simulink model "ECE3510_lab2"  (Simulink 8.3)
settings: Solver=ode1  StartTime=0.0  StopTime=Inf  FixedStep=Ts  RelTol=1e-3
PostLoadFcn:
  | , if any(exist('dsrtsu_mdlpostloadfcn', 'file') == [2, 3, 6]), try dsrtsu_mdlpostloadfcn('Execute', bdroot); catch fprintf('Error in PostLoadFcn (dsrtsu_mdlpostloadfcn) for model "%s":
  |  %s
  | ', bdroot, lasterr); end, end,
InitFcn:
  | Ts=1e-4;
  | nd=30;
libraries: rtilib1104 x4

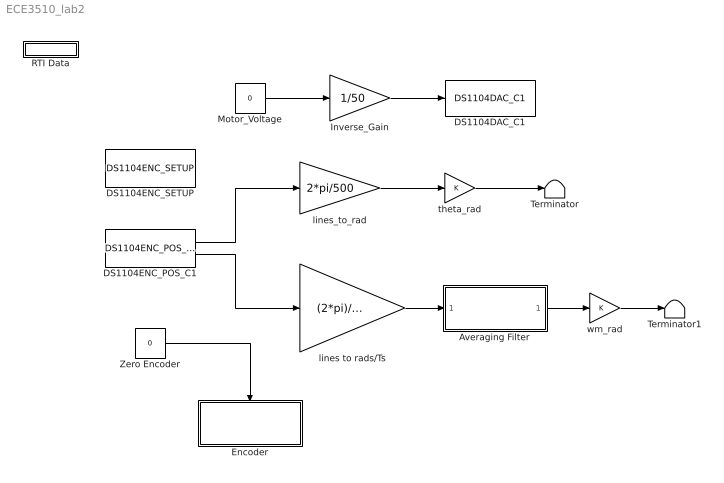
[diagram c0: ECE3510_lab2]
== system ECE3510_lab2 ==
  Averaging Filter : Subsystem
  DS1104DAC_C1 : rtilib1104/DS1104 MASTER PPC/DS1104DAC_C1  ChannelNo=1  InitValue=0  TermMode=0  TermValue=0  Reserved1=[]  Reserved2=[]  Reserved3=[]  Reserved4=[]  DialogFcn=gui1104dac  UnitName={ 'DS1104DAC_C'}  UnitValues={ 1 }  DSProperties=struct('RTI',struct('Version',uint32(1),'BlockType',struct('isSLSource',uint8(0),'isSLSink',uint8(1),'isHWSource',uint8(0),'isHWSink',uint8(1),'isSetup',uint8(0),'isInline',uint8(1),'isNonInline',uint8(0),'isInterrupt',uint8(0),'isChannelwise',uint8(1)),'IOBoardType','DS1104MASTER','UnitType','DAC','Identifier','DAC','DialogType','ML','BlockSet','NONE','SlaveProcessor','NONE'))
  DS1104ENC_POS_C1 : rtilib1104/DS1104 MASTER PPC/DS1104ENC_POS_C1  ChannelNo=1  PosValue=0  Reserved1=[]  Reserved2=[]  Reserved3=[]  Reserved4=[]  DialogFcn=gui1104enc_pos  UnitName={'DS1104ENC_POS_C'}  UnitValues={ 1 }  DSProperties=struct('RTI',struct('Version',uint32(1),'BlockType',struct('isSLSource',uint8(1),'isSLSink',uint8(0),'isHWSource',uint8(1),'isHWSink',uint8(0),'isSetup',uint8(0),'isInline',uint8(1),'isNonInline',uint8(0),'isInterrupt',uint8(0),'isChannelwise',uint8(1)),'IOBoardType','DS1104MASTER','UnitType','ENC','Identifier','ENCPOSCH','DialogType','ML','BlockSet','NONE','SlaveProcessor','NONE'))
  DS1104ENC_SETUP : rtilib1104/DS1104 MASTER PPC/DS1104ENC_SETUP  Reserved1=[]  Reserved2=[]  Reserved3=[]  Reserved4=[]  DialogFcn=gui1104enc_setup  UnitName={'DS1104ENC_SETUP'}  UnitValues={ [] }  DSProperties=struct('RTI',struct('Version',uint32(1),'BlockType',struct('isSLSource',uint8(0),'isSLSink',uint8(0),'isHWSource',uint8(0),'isHWSink',uint8(0),'isSetup',uint8(0),'isInline',uint8(1),'isNonInline',uint8(0),'isInterrupt',uint8(0),'isChannelwise',uint8(0)),'IOBoardType','DS1104MASTER','UnitType','ENC','Identifier','ENCSETUP','DialogType','ML','BlockSet','NONE','SlaveProcessor','NONE'))
  Encoder : Subsystem
  Inverse_Gain : Gain  Gain=1/50
  Motor_Voltage : Constant  Value=0
  RTI Data : Subsystem  Tag=struct('RTIDataServer',struct('RTIDataServerVs','2','RTIModelDescription','struct(''main'',''ECE3510_lab2'',''sub'','''',''isMp'',0)'))  LoadFcn="if exist('rtidc'), try,  rtidc('DataHostBlockClbLoad', gcbh); catch, disp(['Warning: ''LoadFcn'' for RTI Data block failed: ' lasterr]); end, end,"
  Terminator : Terminator
  Terminator1 : Terminator
  Zero Encoder : Constant  Value=0
  lines to rads/Ts : Gain  Gain=(2*pi)/(500*Ts)
  lines_to_rad : Gain  Gain=2*pi/500
  theta_rad : Gain
  wm_rad : Gain
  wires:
  Motor_Voltage/1 -> Inverse_Gain/1
  Inverse_Gain/1 -> DS1104DAC_C1/1
  wm_rad/1 -> Terminator1/1
  theta_rad/1 -> Terminator/1
  lines_to_rad/1 -> theta_rad/1
  Averaging Filter/1(Out1) -> wm_rad/1
  lines to rads/Ts/1 -> Averaging Filter/1(In1)
  DS1104ENC_POS_C1/2 -> lines to rads/Ts/1
  DS1104ENC_POS_C1/1 -> lines_to_rad/1
  Zero Encoder/1 -> Encoder/Trigger

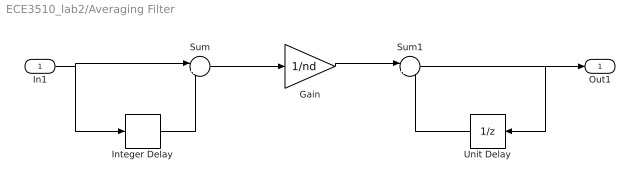
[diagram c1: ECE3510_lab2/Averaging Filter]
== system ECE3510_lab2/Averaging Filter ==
  In1 : Inport
  Gain : Gain  Gain=1/nd
  Integer Delay : Delay  DelayLength=nd
  Sum : Sum  Inputs=|+-
  Sum1 : Sum  Inputs=|++
  Unit Delay : UnitDelay  SampleTime=-1
  Out1 : Outport
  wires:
  In1/1 -> Sum/1, Integer Delay/1
  Integer Delay/1 -> Sum/2
  Sum/1 -> Gain/1
  Gain/1 -> Sum1/1
  Sum1/1 -> Out1/1, Unit Delay/1
  Unit Delay/1 -> Sum1/2

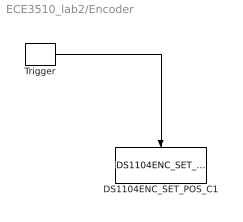
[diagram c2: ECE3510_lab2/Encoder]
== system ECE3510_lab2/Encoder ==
  Trigger : TriggerPort  TriggerType=either  ShowOutputPort=on
  DS1104ENC_SET_POS_C1 : rtilib1104/DS1104 MASTER PPC/DS1104ENC_SET_POS_C1  ChannelNo=1  PosValue=0  Reserved1=[]  Reserved2=[]  Reserved3=[]  Reserved4=[]  DialogFcn=gui1104enc_set_pos  UnitName={'DS1104ENC_SET_POS_C'}  UnitValues={ 1 }  DSProperties=struct('RTI',struct('Version',uint32(1),'BlockType',struct('isSLSource',uint8(0),'isSLSink',uint8(1),'isHWSource',uint8(0),'isHWSink',uint8(1),'isSetup',uint8(0),'isInline',uint8(1),'isNonInline',uint8(0),'isInterrupt',uint8(0),'isChannelwise',uint8(1)),'IOBoardType','DS1104MASTER','UnitType','ENC','Identifier','ENCRESET','DialogType','ML','BlockSet','NONE','SlaveProcessor','NONE'))
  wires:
  Trigger/1 -> DS1104ENC_SET_POS_C1/Trigger

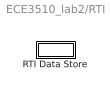
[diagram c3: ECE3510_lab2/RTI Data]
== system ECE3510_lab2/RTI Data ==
  RTI Data Store : Subsystem  Tag=struct('private',struct('version',struct('dsVer',uint32(2),'dsVerCreation',uint32(2),'RTI',struct('ver','7.2','type','RTI1104')),'access',struct('type','Model','isPerm',1,'created',['18-Jan-2017 11:46:42'],'modified',['19-Jan-2017 18:13:45'],'location','')),'public',struct('main',struct('data',[]),'sub',struct('name',{{'ECE3510_lab2'}},'data',{{struct('TH',struct('thTaskInfo',struct('taskType',{'T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

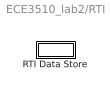
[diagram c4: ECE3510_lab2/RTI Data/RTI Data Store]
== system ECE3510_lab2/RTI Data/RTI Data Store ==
  RTI Data Store : Subsystem

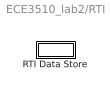
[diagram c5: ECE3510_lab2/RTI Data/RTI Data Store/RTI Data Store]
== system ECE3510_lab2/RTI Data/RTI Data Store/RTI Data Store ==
  RTI Data Store : Subsystem

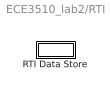
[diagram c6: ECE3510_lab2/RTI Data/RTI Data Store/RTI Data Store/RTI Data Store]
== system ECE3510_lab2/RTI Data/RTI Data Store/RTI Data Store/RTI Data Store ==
  RTI Data Store : Subsystem

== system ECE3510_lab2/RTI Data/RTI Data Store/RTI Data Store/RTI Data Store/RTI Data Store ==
